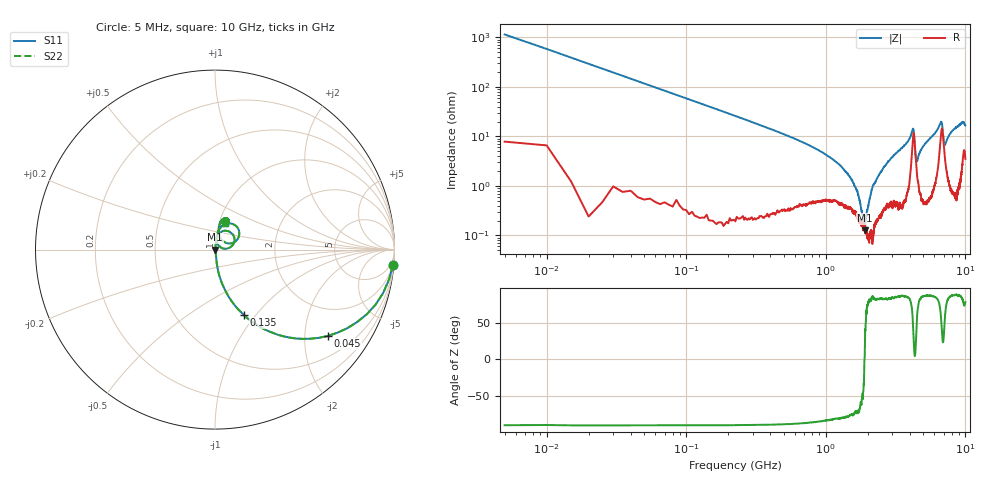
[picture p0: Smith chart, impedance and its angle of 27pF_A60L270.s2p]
! Amotech Co.,Ltd.
! http://www.amotech.co.kr/
! Part Number: A60L270
! These Parameters are Measured in Series Mode Connection
! Operation Temp=25[degC], DC Bias Voltage=0[V]
! Freq. Start=5[MHz] Stop=10[GHz], 2000[Steps]
! Date: Monday, July 14, 2020, 09:40:09
# GHZ S RI R 50.000000
!Freq.(Hz) S11(Real) S11(Imag) S21(Real) S21(Imag) S12(Real) S12(Imag) S22(Real) S22(Imag)
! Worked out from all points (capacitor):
!   2000 points, 5 MHz to 10 GHz, reference 50 ohm
!   read as one part in series: C = 27 pF near 55 MHz
!   lowest |Z| = 128 mohm at 1.9 GHz (marker M1)
!   series resonance near 1.893 GHz, so ESL is about 260 pH
!   S11 on the Smith chart (normalised r, x): 5 MHz: 1, -23; 45 MHz: 1.01, -2.61; 135 MHz: 1.00, -0.87; 10 GHz: 1.07, +0.33
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0.005  0.9919 -0.0863  0.0081 0.0863  0.0081 0.0863  0.9919 -0.0863
0.045  0.6303 -0.4805  0.3697 0.4805  0.3697 0.4805  0.6303 -0.4805
0.075  0.3809 -0.483  0.6191 0.483  0.6191 0.483  0.3809 -0.483
0.135  0.1606 -0.3645  0.8394 0.3645  0.8394 0.3645  0.1606 -0.3645
0.515  0.0145 -0.1054  0.9855 0.1054  0.9855 0.1054  0.0145 -0.1054
1.285  0.00516 -0.0243  0.9948 0.0243  0.9948 0.0243  0.00516 -0.0243
1.675  0.00275 -0.00752  0.9972 0.00752  0.9972 0.00752  0.00275 -0.00752
1.9  0.00128 8.71e-05  0.9987 -8.71e-05  0.9987 -8.71e-05  0.00128 8.71e-05
2.095  0.00126 0.0064  0.9987 -0.0064  0.9987 -0.0064  0.00126 0.0064
2.21  0.00123 0.0107  0.9988 -0.0107  0.9988 -0.0107  0.00123 0.0107
2.615  0.00389 0.0241  0.9961 -0.0241  0.9961 -0.0241  0.00389 0.0241
3.34  0.00655 0.0511  0.9934 -0.0511  0.9934 -0.0511  0.00655 0.0511
4.2  0.089 0.0942  0.911 -0.0942  0.911 -0.0942  0.089 0.0942
4.27  0.1058 0.0374  0.8942 -0.0374  0.8942 -0.0374  0.1058 0.0374
4.4  0.0371 0.00934  0.9629 -0.00934  0.9629 -0.00934  0.0371 0.00934
4.47  0.0218 0.0221  0.9782 -0.0221  0.9782 -0.0221  0.0218 0.0221
5.005  0.00837 0.0633  0.9916 -0.0633  0.9916 -0.0633  0.00837 0.0633
6.67  0.1105 0.1365  0.8895 -0.1365  0.8895 -0.1365  0.1105 0.1365
7.105  0.0421 0.0489  0.9579 -0.0489  0.9579 -0.0489  0.0421 0.0489
8.335  0.0259 0.1369  0.9741 -0.1369  0.9741 -0.1369  0.0259 0.1369
9.57  0.0646 0.1758  0.9354 -0.1758  0.9354 -0.1758  0.0646 0.1758
10  0.0577 0.1491  0.9423 -0.1491  0.9423 -0.1491  0.0577 0.1491
